(* Logix 5000 DataType export PF_Parameters; software revision 32.01 *)

TYPE PF_Parameters :
STRUCT
   ADR_1A : SINT;
   ADR_2A : SINT;
   ADR_3A : SINT;
   ADR_4A : SINT;
   ADR_5A : SINT;
   ADR_6A : SINT;
   ADR_7A : SINT;
   ADR_8A : SINT;
   ADR_9A : SINT;
   ADR_10A : SINT;
   ADR_11A : SINT;
   ADR_12A : SINT;
   ADR_13A : SINT;
   ADR_14A : SINT;
   ADR_15A : SINT;
   ADR_16A : SINT;
   ADR_17A : SINT;
   ADR_18A : SINT;
   ADR_19A : SINT;
   ADR_20A : SINT;
   ADR_21A : SINT;
   ADR_22A : SINT;
   ADR_23A : SINT;
   ADR_24A : SINT;
   ADR_25A : SINT;
   ADR_26A : SINT;
   ADR_27A : SINT;
   ADR_28A : SINT;
   ADR_29A : SINT;
   ADR_30A : SINT;
   ADR_31A : SINT;
   ADR_1B : SINT;
   ADR_2B : SINT;
   ADR_3B : SINT;
   ADR_4B : SINT;
   ADR_5B : SINT;
   ADR_6B : SINT;
   ADR_7B : SINT;
   ADR_8B : SINT;
   ADR_9B : SINT;
   ADR_10B : SINT;
   ADR_11B : SINT;
   ADR_12B : SINT;
   ADR_13B : SINT;
   ADR_14B : SINT;
   ADR_15B : SINT;
   ADR_16B : SINT;
   ADR_17B : SINT;
   ADR_18B : SINT;
   ADR_19B : SINT;
   ADR_20B : SINT;
   ADR_21B : SINT;
   ADR_22B : SINT;
   ADR_23B : SINT;
   ADR_24B : SINT;
   ADR_25B : SINT;
   ADR_26B : SINT;
   ADR_27B : SINT;
   ADR_28B : SINT;
   ADR_29B : SINT;
   ADR_30B : SINT;
   ADR_31B : SINT;
END_STRUCT
END_TYPE
